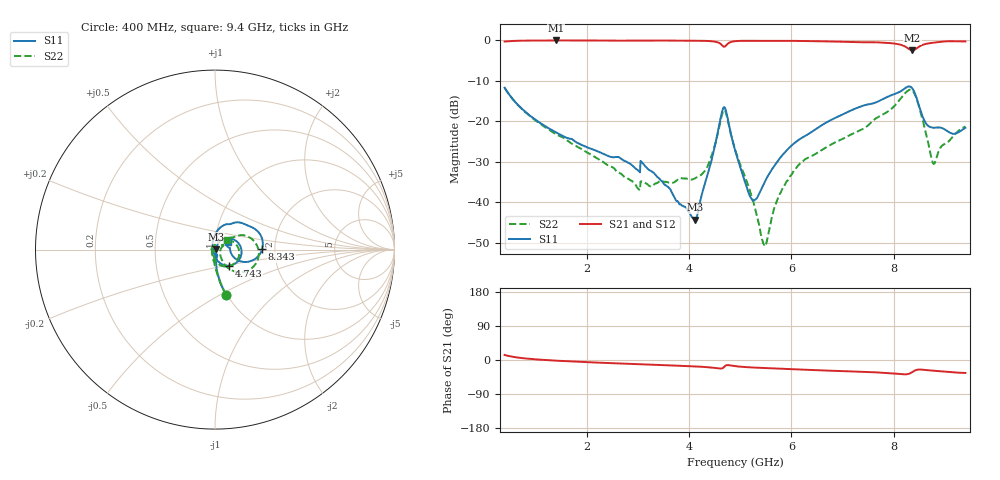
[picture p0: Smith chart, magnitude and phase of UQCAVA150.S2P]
!  Part Number  UQCAVA150
!  Description: RF capacitor  Mounting Orientation: Horizontal
!  Application:
# GHZ S DB R 50
! Freq  |S11|  S11 Ph  |S21|  S21 Ph  |S12|  S12 Ph  |S22|  S22 Ph
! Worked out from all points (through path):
!   801 points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, 400 MHz to 9.4 GHz, reference 50 ohm
!   highest |S21| = -0.06 dB at 1.401 GHz (marker M1); lowest = -2.5 dB at 8.365 GHz (marker M2)
!   group delay of S21, straight-line fit = 12.4 ps
!   lowest |S11| = -44.3 dB at 4.124 GHz (marker M3), VSWR 1.01, Z = 50.6 + j0.166 ohm
!   |S11| at or under -10 dB: start of sweep to end of sweep
!   |S22| runs from -50.8 to -11.7 dB; largest |S21 - S12| = 0.0019
!   S11 on the Smith chart (normalised r, x): 400 MHz: 0.99, -0.53; 4.743 GHz: 1.15, -0.21; 8.343 GHz: 1.71, +0.02; 9.4 GHz: 1.15, +0.10
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0.4  -11.72 -76.3  -0.32 13.3  -0.32 13.3  -11.73 -76.1
1.401  -22.71 -85.2  -0.06 -1.7  -0.06 -1.7  -23.14 -94.3
1.908  -25.83 -81.3  -0.07 -5.1  -0.06 -5.1  -26.87 -105.7
2.999  -32.00 -70.6  -0.13 -10.8  -0.13 -10.9  -36.48 -166.6
3.1  -30.34 -81.2  -0.12 -11.2  -0.11 -11.3  -34.94 -147.9
3.404  -33.94 -76.8  -0.09 -12.9  -0.08 -12.9  -35.01 -147.2
4.124  -44.26 15.5  -0.14 -17.0  -0.14 -17.1  -34.02 133.3
4.383  -32.31 63.9  -0.20 -19.2  -0.19 -19.3  -30.51 88.2
4.641  -17.90 22.4  -1.17 -22.3  -1.16 -22.3  -18.59 17.3
4.743  -18.41 -47.9  -1.06 -13.6  -1.06 -13.6  -18.88 -56.1
4.9  -27.06 -86.9  -0.24 -16.2  -0.23 -16.2  -26.88 -97.0
5.226  -39.20 -155.8  -0.13 -19.6  -0.13 -19.7  -38.42 -109.0
5.474  -35.15 134.0  -0.15 -21.2  -0.15 -21.3  -50.70 -41.4
5.856  -27.89 109.1  -0.15 -23.3  -0.15 -23.3  -36.04 34.6
6.408  -22.51 92.7  -0.23 -26.4  -0.23 -26.4  -28.49 30.9
7.904  -13.82 47.9  -0.69 -34.5  -0.70 -34.6  -17.43 32.8
8.343  -11.59 1.1  -2.46 -33.5  -2.46 -33.5  -12.24 -14.0
8.365  -11.90 -4.4  -2.50 -31.6  -2.51 -31.6  -12.43 -20.3
8.601  -19.88 -18.4  -0.99 -26.1  -1.00 -26.1  -21.47 -57.3
8.781  -21.57 1.8  -0.60 -28.2  -0.61 -28.3  -30.49 -12.1
8.95  -21.68 6.9  -0.35 -29.9  -0.36 -29.9  -25.92 24.2
9.4  -21.59 30.5  -0.30 -34.2  -0.31 -34.3  -21.29 38.0
